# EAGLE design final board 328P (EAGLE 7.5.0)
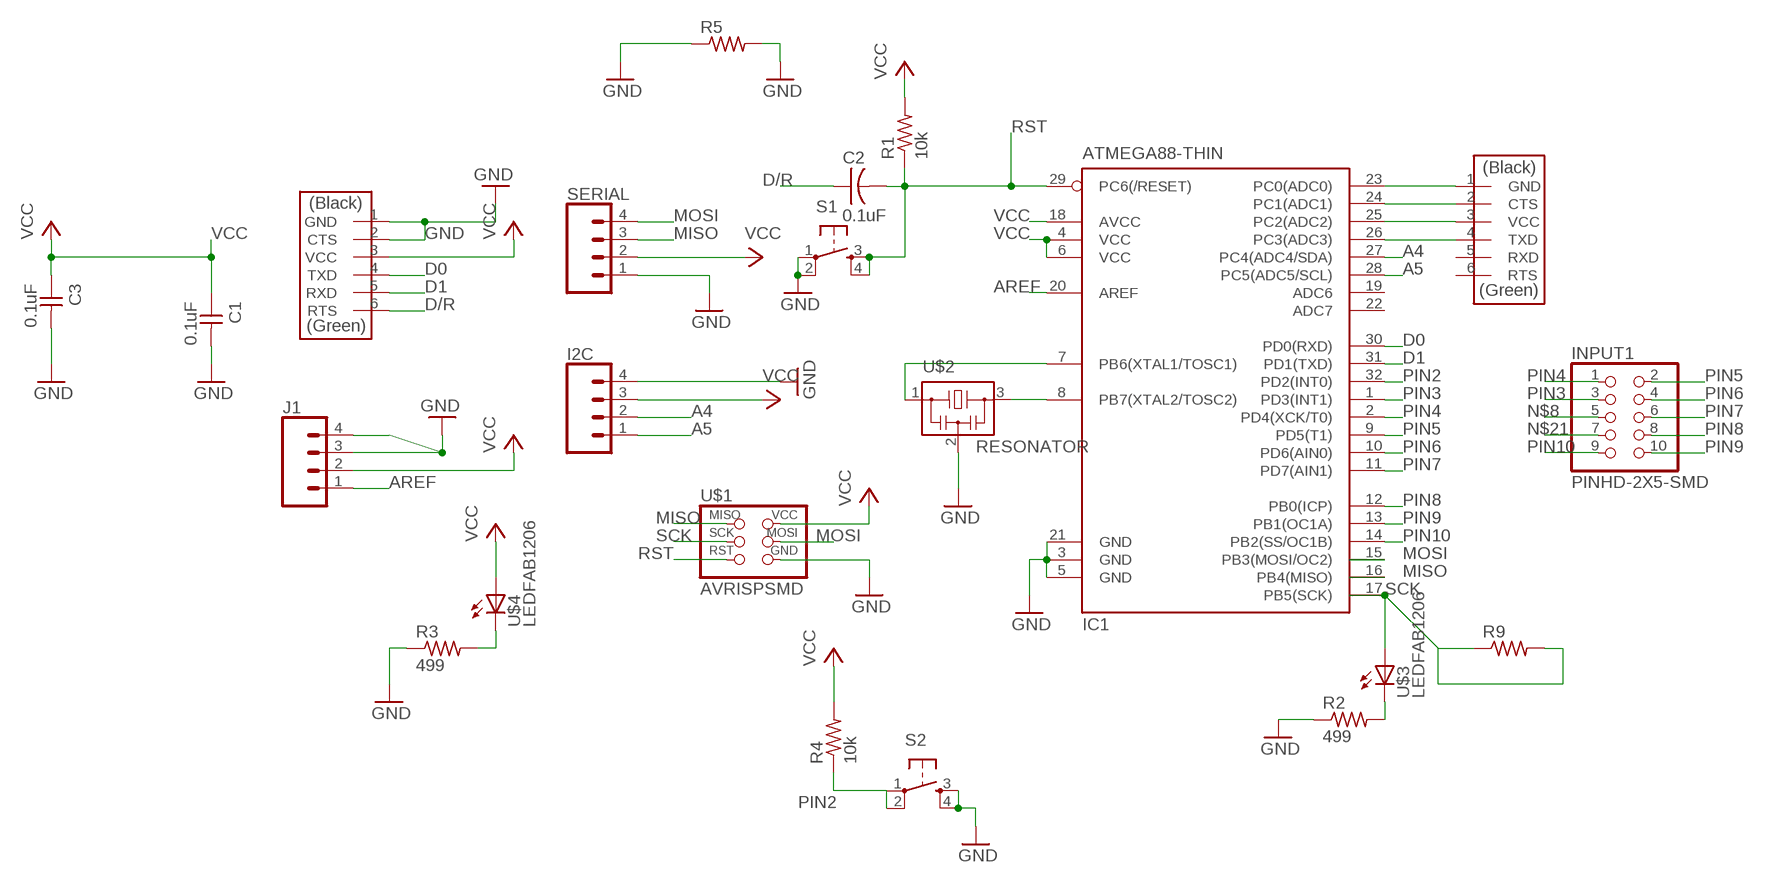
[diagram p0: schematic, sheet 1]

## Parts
C1  0.1uF  CAP-UNPOLARIZEDFAB  [C1206FAB]
C2  0.1uF  CAP-US1206FAB  [C1206FAB]
C3  0.1uF  CAP-UNPOLARIZEDFAB  [C1206FAB]
I2C  CONN_04SMD  [1X04_SMD_RA_MALE]
IC1  ATMEGA88-THIN  [TQFP32-08THIN]
INPUT1  PINHD-2X5-SMD  [2X05SMD]
J1  CONN_04SMD  [1X04_SMD_RA_MALE]
R1  10k  RES-US1206FAB  [R1206FAB]
R2  499  RES-US1206FAB  [R1206FAB]
R3  499  RES-US1206FAB  [R1206FAB]
R4  10k  RES-US1206FAB  [R1206FAB]
R5  RES-US1206FAB  [R1206FAB]
R9  RES-US1206FAB  [R1206FAB]
S1  6MM_SWITCH6MM_SWITCH  [6MM_SWITCH]
S2  6MM_SWITCH6MM_SWITCH  [6MM_SWITCH]
SERIAL  CONN_04SMD  [1X04_SMD_RA_MALE]
U$1  AVRISPSMD  [2X03SMD]
U$2  RESONATOR  [EFOBM]
U$3  LEDFAB1206  [LED1206FAB]
U$4  LEDFAB1206  [LED1206FAB]
U$5  FTDI-SMD-HEADER  [1X06SMD]
U$6  FTDI-SMD-HEADER  [1X06SMD]

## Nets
A4: I2C.2 IC1.27(PC4(ADC4/SDA))
A5: I2C.1 IC1.28(PC5(ADC5/SCL))
AREF: IC1.20(AREF) J1.1
D0: IC1.30(PD0(RXD)) U$6.4(TXD)
D1: IC1.31(PD1(TXD)) U$6.5(RXD)
D/R: C2.1 U$6.6(RTS)
GND: C1.2 C3.2 I2C.4 IC1.3(GND) IC1.5(GND) IC1.21(GND) J1.3 J1.4 R2.1 R3.1 R5.1 R5.2 S1.1(P) S1.2(P1) S2.3(S) S2.4(S1) SERIAL.1 U$1.6(GND) U$2.2 U$6.1(GND) U$6.2(CTS)
MISO: IC1.16(PB4(MISO)) SERIAL.3 U$1.1(MISO)
MOSI: IC1.15(PB3(MOSI/OC2)) SERIAL.4 U$1.4(MOSI)
N$1: IC1.23(PC0(ADC0)) U$5.1(GND)
N$2: IC1.24(PC1(ADC1)) U$5.2(CTS)
N$3: IC1.25(PC2(ADC2)) U$5.3(VCC)
N$4: IC1.26(PC3(ADC3)) U$5.4(TXD)
N$8: INPUT1.5
N$11: IC1.8(PB7(XTAL2/TOSC2)) U$2.3
N$12: IC1.7(PB6(XTAL1/TOSC1)) U$2.1
N$13: R2.2 U$3.2(C)
N$14: R3.2 U$4.2(C)
N$21: INPUT1.7
PIN2: IC1.32(PD2(INT0)) R4.1 S2.1(P) S2.2(P1)
PIN3: IC1.1(PD3(INT1)) INPUT1.3
PIN4: IC1.2(PD4(XCK/T0)) INPUT1.1
PIN5: IC1.9(PD5(T1)) INPUT1.2
PIN6: IC1.10(PD6(AIN0)) INPUT1.4
PIN7: IC1.11(PD7(AIN1)) INPUT1.6
PIN8: IC1.12(PB0(ICP)) INPUT1.8
PIN9: IC1.13(PB1(OC1A)) INPUT1.10
PIN10: IC1.14(PB2(SS/OC1B)) INPUT1.9
RST: C2.2 IC1.29(PC6(/RESET)) R1.1 S1.3(S) S1.4(S1) U$1.5(RST)
SCK: IC1.17(PB5(SCK)) R9.1 R9.2 U$1.3(SCK) U$3.1(A)
VCC: C1.1 C3.1 I2C.3 IC1.4(VCC) IC1.6(VCC) IC1.18(AVCC) J1.2 R1.2 R4.2 SERIAL.2 U$1.2(VCC) U$4.1(A) U$6.3(VCC)
Unconnected: IC1.19(ADC6) IC1.22(ADC7) U$5.5(RXD) U$5.6(RTS)

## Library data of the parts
C1 C3 = fab:CAP-UNPOLARIZED
C2 = fab:CAP-US
I2C J1 SERIAL = SparkFun-Connectors:CONN_04: Multi connection point. Often used as Generic Header-pin footprint for 0.1 inch spaced/style header connections On any of the 0.1 inch spaced packages, you can populate with these: Break Away Headers - Straight (PRT-00116) Break Away Male Headers - Right Angle (PRT-00553) Female Headers (PRT-00115)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; PROD_ID: CONN-09140; SF_ID: PRT-12638
IC1 = fab:ATMEGA88-THIN
INPUT1 = fab:PINHD-2X5-SMD
R1-R5 R9 = fab:RES-US: Resistor (US Symbol)
S1 S2 = fab:6MM_SWITCH: OMRON SWITCH
U$1 = fab:AVRISP
U$2 = fab:RESONATOR
U$3 U$4 = fab:LED: LED
U$5 U$6 = fab:FTDI-SMD-HEADER

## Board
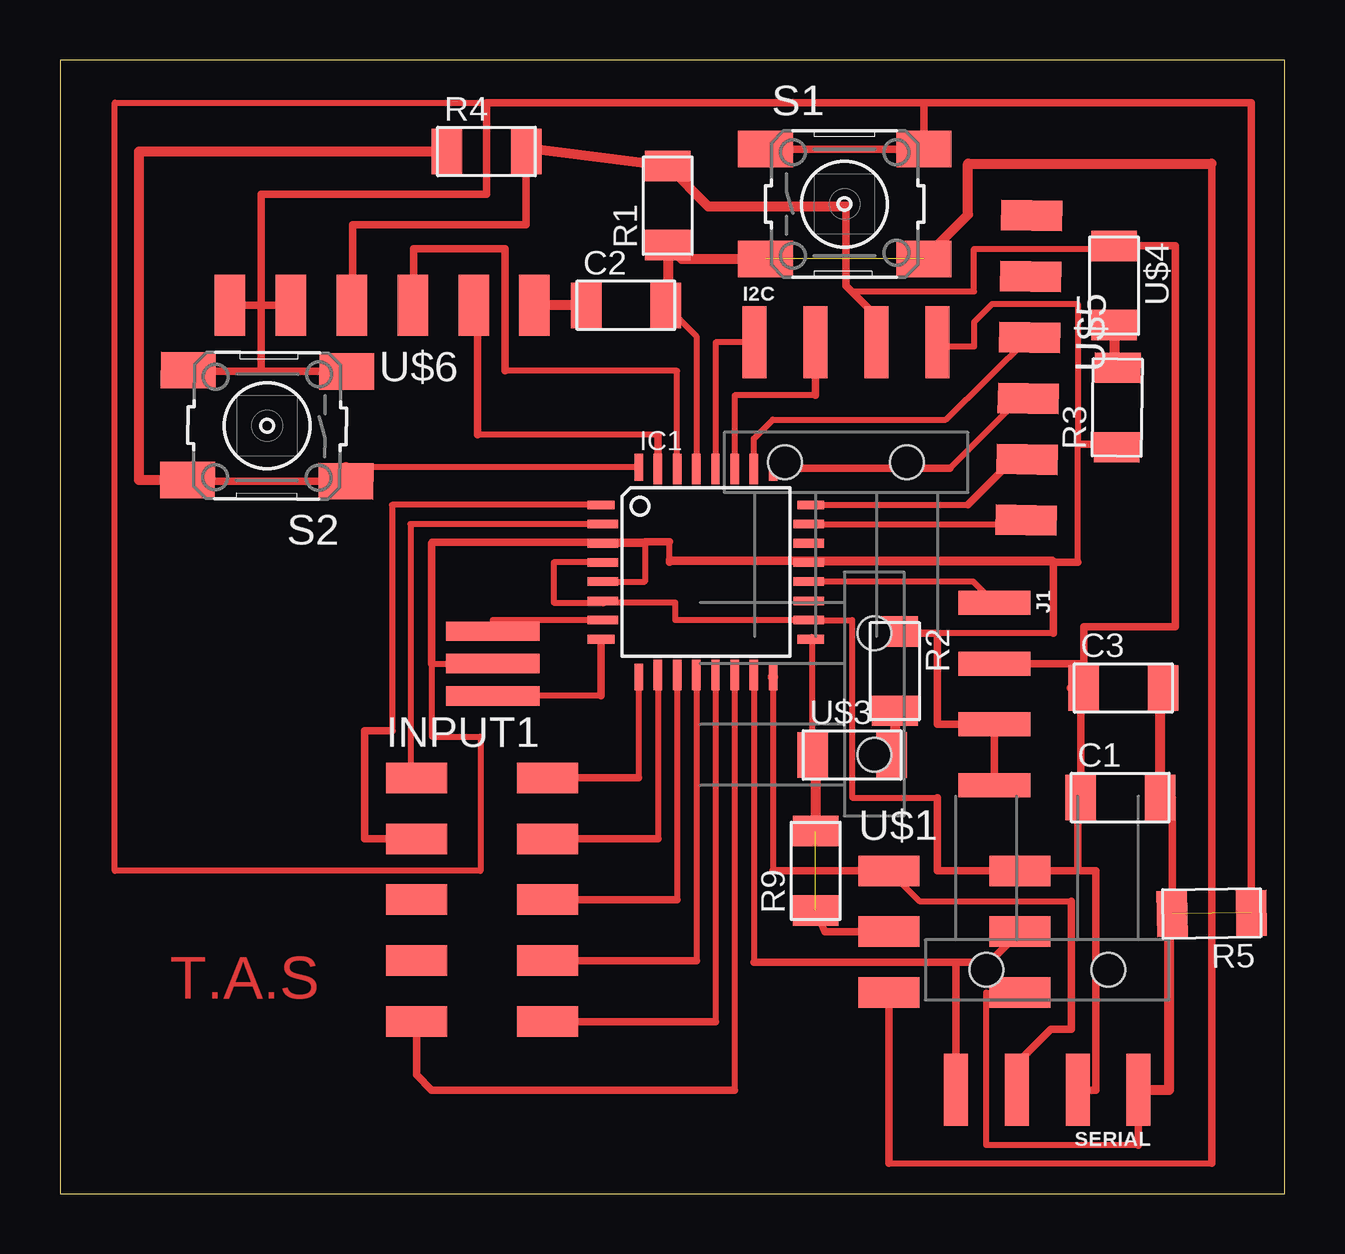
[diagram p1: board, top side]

Size 51.05 x 47.24 mm. Coordinates in mm from the lower left corner, seen from the top.
Outline: 0,0 51.05,0 51.05,47.24 0,47.24 0,0
Copper layers (1*16): Top 0.035mm / dielectric 1.5mm / Bottom 0.035mm
Design rules "default *": minimum track width 10mil, minimum drill 24mil, track to track 16mil, track to pad 8mil, pad to pad 8mil, via to via 8mil, smd to smd 8mil, copper to edge 40mil, drill to drill 8mil, minimum pad ring 10mil, minimum via ring 8mil, stop-mask expansion 4mil, vias tented up to drill 0mil, thermal gap 10mil

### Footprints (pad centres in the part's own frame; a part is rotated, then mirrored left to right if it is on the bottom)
C1206FAB = smd 1.27 x 1.905: 1 -1.651,0; 2 1.651,0
1X04_SMD_RA_MALE = smd 1 x 3: 1 -3.81,5; 2 -1.27,5; 3 1.27,5; 4 3.81,5 | hole 1.4: -2.54,0; 2.54,0
TQFP32-08THIN = smd 1.118 x 0.356: 1 -4.369,2.8; 8 -4.369,-2.8; 17 4.369,-2.8; 24 4.369,2.8 | smd 1.27 x 0.356: 2 -4.293,2; 3 -4.293,1.2; 4 -4.293,0.4; 5 -4.293,-0.4; 6 -4.293,-1.2; 7 -4.293,-2; 18 4.293,-2; 19 4.293,-1.2; 20 4.293,-0.4; 21 4.293,0.4; 22 4.293,1.2; 23 4.293,2 | smd 0.356 x 1.118: 9 -2.8,-4.369; 16 2.8,-4.369; 25 2.8,4.369; 32 -2.8,4.369 | smd 0.356 x 1.27: 10 -2,-4.293; 14 1.2,-4.293; 15 2,-4.293; 26 2,4.293; 27 1.2,4.293; 31 -2,4.293 | smd 0.35 x 1.27: 11 -1.2,-4.293; 12 -0.4,-4.293; 13 0.4,-4.293; 28 0.4,4.293; 29 -0.4,4.293; 30 -1.2,4.293
2X05SMD = smd 2.54 x 1.27: 1 -2.54,2.54; 2 2.92,2.54; 3 -2.54,0; 4 2.92,0; 5 -2.54,-2.54; 6 2.92,-2.54; 7 -2.54,-5.08; 8 2.92,-5.08; 9 -2.54,-7.62; 10 2.92,-7.62
R1206FAB = smd 1.27 x 1.905: 1 -1.651,0; 2 1.651,0
6MM_SWITCH = smd 2.286 x 1.524: 1 -3.302,2.286; 2 3.302,2.286; 3 -3.302,-2.286; 4 3.302,-2.286
2X03SMD = smd 2.54 x 1.27: 1 -2.54,2.54; 2 2.92,2.54; 3 -2.54,0; 4 2.92,0; 5 -2.54,-2.54; 6 2.92,-2.54
EFOBM = smd 0.8 x 3.9: 1 -1.35,0; 2 0,0; 3 1.35,0
LED1206FAB = smd 1.27 x 1.905: 1 -1.651,0; 2 1.651,0
1X06SMD = smd 2.54 x 1.27: 1 0,6.35; 2 0,3.81; 3 0,1.27; 4 0,-1.27; 5 0,-3.81; 6 0,-6.35

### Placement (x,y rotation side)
C1  44.2,16.51 0 top
C2  23.59,37.02 0 top
C3  44.32,21.08 0 top
I2C  32.77,30.48 0 top
IC1  26.92,25.91 0 top
INPUT1  17.4,14.8 0 top
J1  33.94,20.83 270 top
R1  25.34,41.18 90 top
R2  34.8,21.78 270 top
R3  44.07,32.77 89.3 top
R4  17.78,43.43 0 top
R5  48.01,11.68 180.8 top
R9  31.5,13.46 90 top
S1  32.7,41.24 0 top
S2  8.64,32 179.6 top
SERIAL  41.15,9.33 180 top
U$1  37.08,10.92 0 top
U$2  18.03,22.1 270 top
U$3  33.02,18.29 0 top
U$4  43.94,37.85 270 top
U$5  40.39,34.42 179 top
U$6  13.43,37.02 90 top

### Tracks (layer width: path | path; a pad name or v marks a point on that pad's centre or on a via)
A4
  Top 0.254: 31.5,33.27 28.12,33.27 IC1.27
  Top 0.305: 31.5,33.27 I2C.2
A5
  Top 0.254: I2C.1 27.32,35.48 IC1.28
AREF
  Top 0.254: IC1.20 38.07,25.51 J1.1
D0
  Top 0.254: IC1.30 25.72,34.29 18.54,34.29
  Top 0.305: 18.54,34.29 18.54,39.37 14.73,39.37 14.73,37.02
  Top 0.406: 14.73,37.02 U$6.4
D1
  Top 0.254: 24.92,31.62 17.4,31.62
  Top 0.305: IC1.31 24.92,31.62 | 17.4,31.62 17.4,37.02
  Top 0.406: 17.4,37.02 U$6.5
D/R
  Top 0.406: C2.1 U$6.6
GND  (1 unrouted)
  Top 0.254: IC1.3 15.49,27.11 | 15.49,22.1 U$2.2 | IC1.5 24.38,25.51 24.38,27.11 | 44.96,2.03 38.61,2.03 38.61,8.38 U$1.6 | 36.58,35.31 38.1,35.31 38.1,36.32 38.86,37.08 42.42,37.08 42.42,31.24 42.42,26.31 | 25.4,26.31 IC1.21 41.4,26.31 | 41.4,23.37 36.58,23.37 | 41.4,26.16 41.4,26.42 25.4,26.42 25.4,27.18 15.49,27.18 15.49,19.05 17.53,19.05 17.53,13.46 2.29,13.46 2.29,45.47 17.78,45.47 | 8.38,34.27 6.1,34.27
  Top 0.305: 15.49,27.11 15.49,22.1 | S1.1 S1.2 36.01,45.47 | IC1.3 24.38,27.11 24.38,27.18 25.4,27.18 | 42.42,31.24 43.43,31.24 | SERIAL.1 44.96,2.03 | 36.58,35.31 I2C.4 | 11.95,34.31 S2.3 6.1,34.27 5.35,34.27 S2.4 | J1.4 J1.3 36.58,19.56 36.58,23.37 34.8,23.37 R2.1 | 25.4,26.31 25.4,26.42 | 42.42,26.31 41.4,26.31 41.4,26.16 41.4,23.37 | U$6.1 8.38,37.02 | 8.38,37.02 8.38,34.27 | 8.38,37.02 8.38,41.66 17.78,41.66 17.78,45.47 36.01,45.47 | 36.01,45.47 49.66,45.47 R5.1 | C1.2 46.35,16.51 R5.2 | U$6.2 8.38,37.02
  Top 0.406: 43.43,31.24 R3.1 | C3.2 45.85,21.08 C1.2 | R5.2 46.23,11.66 46.23,4.32 44.96,4.32 SERIAL.1
MISO
  Top 0.254: IC1.16 29.72,13.46 | U$1.1 35.81,12.19 42.16,12.19
  Top 0.305: 29.72,13.46 U$1.1 | 42.16,12.19 42.16,6.86 41.31,6.86 39.69,5.25
  Top 0.406: SERIAL.3 39.69,5.25 39.62,5.59 | IC1.16
MOSI
  Top 0.254: IC1.15 28.92,9.65
  Top 0.305: 28.92,9.65 37.34,9.65 | 37.34,9.65 38.73,9.65 U$1.4 | SERIAL.4 37.34,9.65
N$1
  Top 0.254: IC1.23 40.56,27.91
  Top 0.406: 40.56,27.91 U$5.1
N$2
  Top 0.254: IC1.24 37.85,28.71
  Top 0.305: 37.85,28.71 39.62,30.48
  Top 0.406: 39.62,30.48 40.36,30.48 U$5.2
N$3
  Top 0.254: 40.01,33.15 37.08,30.23
  Top 0.305: 37.08,30.23 29.77,30.23
  Top 0.406: U$5.3 40.01,33.15 | 29.77,30.23 IC1.25
N$4
  Top 0.254: IC1.26 28.92,31.46 29.72,32.26 36.92,32.26 U$5.4
N$11
  Top 0.254: 22.55,20.75 U$2.3
  Top 0.305: IC1.8 22.55,20.75
N$12
  Top 0.254: IC1.7 18.03,23.91 U$2.1
N$13
  Top 0.406: R2.2 34.8,18.29 U$3.2
N$14
  Top 0.406: U$4.2 43.94,34.42 R3.2
PIN2
  Top 0.254: IC1.32 11.92,30.28
  Top 0.305: S2.2 5.32,29.7 S2.1
  Top 0.406: S2.2 3.3,29.74 3.3,43.43 R4.1 | 11.92,30.28 S2.1
PIN3
  Top 0.254: IC1.1 13.84,28.71 13.84,19.3
  Top 0.305: 13.84,19.3 12.7,19.3 12.7,14.8 INPUT1.3
  Top 0.406: 14.86,14.48 INPUT1.3
PIN4
  Top 0.254: IC1.2 14.61,27.91 14.61,17.34
  Top 0.406: 14.61,17.34 INPUT1.1
PIN5
  Top 0.254: IC1.9 24.12,17.34
  Top 0.305: 24.12,17.34 INPUT1.2
PIN6
  Top 0.254: IC1.10 24.92,14.8
  Top 0.305: 24.92,14.8 INPUT1.4
PIN7
  Top 0.254: IC1.11 25.72,12.26
  Top 0.305: 25.72,12.26 INPUT1.6
PIN8
  Top 0.254: IC1.12 26.52,9.72
  Top 0.305: 26.52,9.72 INPUT1.8
PIN9
  Top 0.254: IC1.13 27.32,7.18
  Top 0.305: 27.32,7.18 INPUT1.10
PIN10
  Top 0.254: IC1.14 28.12,4.32
  Top 0.305: 28.12,4.32 15.49,4.32 14.86,4.95 INPUT1.9
RST  (1 unrouted)
  Top 0.254: C2.2 26.52,35.74 IC1.29 | 34.54,1.27 48.01,1.27
  Top 0.305: 48.01,42.93 48.01,1.27 | U$1.5 34.54,1.27
  Top 0.406: C2.2 25.34,37.02 R1.1 25.91,38.96 S1.3 | S1.4 37.85,40.8 37.85,42.93 48.01,42.93
SCK  (1 unrouted)
  Top 0.254: U$3.1 31.37,23.11
  Top 0.305: R9.1 31.88,10.92 U$1.3
  Top 0.406: 31.37,23.11 IC1.17 | U$3.1 31.5,18.29 R9.2
VCC
  Top 0.254: IC1.4 20.57,26.31 20.57,24.64 22.63,24.64 25.65,24.64 25.65,23.91 IC1.18 33.02,23.91 33.02,16.51 36.58,16.51 | 33.15,37.47 33.02,37.59 38.1,37.59 38.1,39.37 43.43,39.37
  Top 0.305: 22.63,24.64 IC1.6 | R4.2 19.43,40.39 12.19,40.39 12.19,37.02 | 32.77,41.15 32.77,37.85 33.02,37.59 34.04,36.58 | 36.58,16.51 36.58,13.46 U$1.2 | 42.67,22.1 42.67,23.62 46.48,23.62 46.48,39.5 U$4.1 | J1.2 42.67,22.1 | 42.67,22.1 C3.1 42.55,21.08 C1.1 | 42.8,15.75 42.42,15.75 42.42,13.46 U$1.2 | U$1.2 43.18,13.46 43.18,4.32 42.42,4.32 SERIAL.2
  Top 0.406: 12.19,37.02 U$6.3 | R4.2 19.43,43.59 R1.2 27.02,41.15 32.77,41.15 | 42.8,15.75 C1.1 42.67,16.51 | U$4.1 43.43,39.5 43.43,39.37 | 42.16,21.08 C3.1 | I2C.3 34.29,36.07 34.04,36.58

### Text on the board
Top: T.A.S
